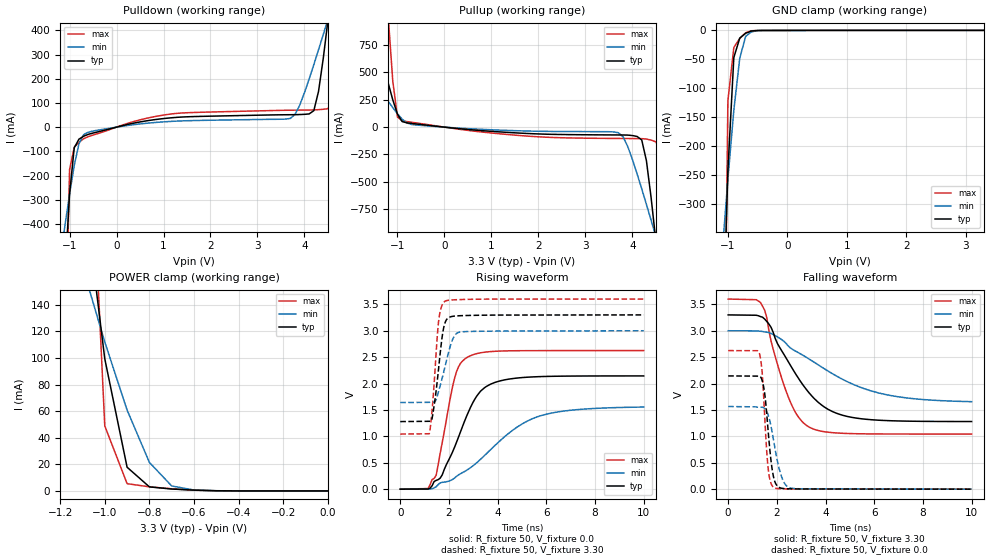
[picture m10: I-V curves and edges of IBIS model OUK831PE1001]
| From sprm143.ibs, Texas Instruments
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[Model]   OUK831PE1001
Model_type   3-state
| INCLUDES PULL DOWN
Enable   Active-Low
Polarity   Non-Inverting
| signals   A, GZ, Y
Vmeas = 1.5
|   typ   min   max
C_comp   2.380p   1.8925p   2.396p
|   typ   min   max
[Temperature Range]   25   -40   125
|   typ   min   max
[Voltage Range]   3.30V   3.00V   3.60V
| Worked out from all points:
|   slope of the pulldown table from 0 to 0.495 V, typ, clamps not added: 23.2 ohm
|   slope of the pullup table from 0 to 0.495 V, typ, clamps not added: 23.3 ohm
|   GND clamp passes 1 mA (typ) near -0.60 V on its own axis
|   POWER clamp passes 1 mA (typ) near -0.65 V on its own axis
|   rising waveform, R_fixture 50, V_fixture 0.0: 20-80 % time 1.22ns typ, 2.49ns min, 650ps max; typ from 0 V to 2.14 V
|   falling waveform, R_fixture 50, V_fixture 3.30: 20-80 % time 1.71ns typ, 3.02ns min, 1.01ns max; typ from 3.3 V to 1.28 V
|   rising waveform, R_fixture 50, V_fixture 3.30: 20-80 % time 302ps typ, 458ps min, 237ps max; typ from 1.28 V to 3.3 V
|   falling waveform, R_fixture 50, V_fixture 0.0: 20-80 % time 266ps typ, 409ps min, 201ps max; typ from 2.15 V to 0 V
[Pulldown]
|   Voltage   I(typ)   I(min)   I(max)
-3.3V     -10.33A    -3.703A    -44.34A
-1.1V     -616.1mA   -409.8mA   -1.053A
-1V       -277.3mA   -277.3mA   -176.2mA
-900mV    -85.21mA   -158.2mA   -82.55mA
-700mV    -37.59mA   -31.02mA   -47.98mA
3.7V      51.31mA    35.94mA    70.02mA
4.1V      54.54mA    198.6mA    70.59mA
4.3V      147.4mA    319.6mA    72.24mA
4.5V      440.5mA    445.2mA    76.18mA
4.6V      607.6mA    508.9mA    117.8mA
4.7V      779.8mA    573.1mA    469.9mA
6.6V      4.227A     1.822A     15.05A
[GND_clamp]
|   Voltage   I(typ)   I(min)   I(max)
-3.3V     -10.32A    -3.701A    -44.29A
-1.1V     -582.7mA   -389.1mA   -1.007A
-1V       -241.9mA   -256.8mA   -121.5mA
-900mV    -46.66mA   -137.5mA   -29.37mA
-800mV    -13.12mA   -47.53mA   -13.83mA
-700mV    -4.697mA   -10.01mA   -4.022mA
-600mV    -940.7uA   -2.307mA   -523.2uA
-400mV    -40.54uA   -69.81uA   -55.88uA
3.3V      100.4uA    53.84uA    176.9uA
[Pullup]
|   Voltage   I(typ)   I(min)   I(max)
-3.3V     4.191A     1.603A     17.37A
-2.3V     2.36A      943.2mA    9.454A
-1.5V     920.2mA    424.9mA    3.222A
-1.2V     406.7mA    238.1mA    1.031A
-1V       118.3mA    122.5mA    92.24mA
-900mV    50.8mA     72.87mA    57.76mA
3.7V      -71.54mA   -51.04mA   -103.5mA
4.2V      -117.2mA   -564.4mA   -105.1mA
4.4V      -646.9mA   -852.4mA   -118.7mA
4.6V      -1.453A    -1.148A    -223.9mA
4.7V      -1.879A    -1.297A    -1.1A
6.6V      -10.33A    -4.164A    -38.3A
[POWER_clamp]
|   Voltage   I(typ)   I(min)   I(max)
-3.3V     4.175A     1.588A     17.36A
-1.1V     235.6mA    168.7mA    405.1mA
-1V       99.35mA    112mA      48.88mA
-900mV    17.82mA    60.81mA    5.459mA
-800mV    3.044mA    21.44mA    3.08mA
-700mV    1.432mA    3.716mA    1.589mA
-600mV    597.6uA    671uA      555.5uA
0V        1pA        1pA        1pA
[Ramp]
|   I(typ)   I(min)   I(max)
dV/dt_r   1.287/1.217n   0.933/2.491n   1.574/0.649n
dV/dt_f   1.212/1.703n   0.806/3.021n   1.534/1.006n
[Rising Waveform]
R_fixture = 50
V_fixture = 0.0
|  pu_on
|  TIME   V(typ)   V(min)   V(max)
0s        3nV        14nV       2nV
1.143ns   3.261mV    14.04nV    11.64mV
1.475ns   166.1mV    46.04mV    262.6mV
2.223ns   785.3mV    207.4mV    2.086V
2.472ns   1.082V     291.7mV    2.38V
2.805ns   1.466V     380.6mV    2.51V
3.303ns   1.858V     567.7mV    2.582V
3.719ns   1.99V      751.1mV    2.605V
5.63ns    2.129V     1.37V      2.623V
10ns      2.144V     1.555V     2.624V
[Falling Waveform]
R_fixture = 50
V_fixture = 3.30
V_fixture_min = 3.00
V_fixture_max = 3.60
|  pd_on
|  TIME   V(typ)   V(min)   V(max)
0s        3.3V       3V         3.6V
1.327ns   3.269V     2.99V      3.536V
1.501ns   3.221V     2.978V     3.386V
1.85ns    2.97V      2.929V     2.65V
2.459ns   2.422V     2.717V     1.759V
2.895ns   2.095V     2.582V     1.361V
3.33ns    1.821V     2.463V     1.175V
5.072ns   1.361V     1.998V     1.052V
6.988ns   1.292V     1.749V     1.044V
10ns      1.28V      1.657V     1.044V
[Rising Waveform]
R_fixture = 50
V_fixture = 3.30
V_fixture_min = 3.00
V_fixture_max = 3.60
|  pd_off
|  TIME   V(typ)   V(min)   V(max)
0s        1.28V      1.641V     1.044V
1.192ns   1.285V     1.644V     1.049V
1.308ns   1.339V     1.65V      1.498V
1.454ns   1.787V     1.676V     2.429V
1.57ns    2.258V     1.845V     3.154V
1.715ns   2.864V     2.089V     3.482V
1.831ns   3.138V     2.304V     3.556V
2.151ns   3.273V     2.836V     3.584V
2.442ns   3.284V     2.974V     3.59V
10ns      3.3V       3V         3.6V
[Falling Waveform]
R_fixture = 50
V_fixture = 0.0
|  pu_off
|  TIME   V(typ)   V(min)   V(max)
0s        2.145V     1.565V     2.624V
1.286ns   2.141V     1.552V     2.568V
1.397ns   2.057V     1.552V     2.21V
1.508ns   1.784V     1.526V     1.312V
1.639ns   1.127V     1.411V     412mV
1.769ns   509.2mV    1.171V     98.84mV
1.899ns   170mV      838.3mV    24.95mV
2.233ns   14.83mV    186.9mV    6.416mV
2.586ns   5.992mV    20.83mV    3.34mV
10ns      1.848uV    60uV       38.11nV
